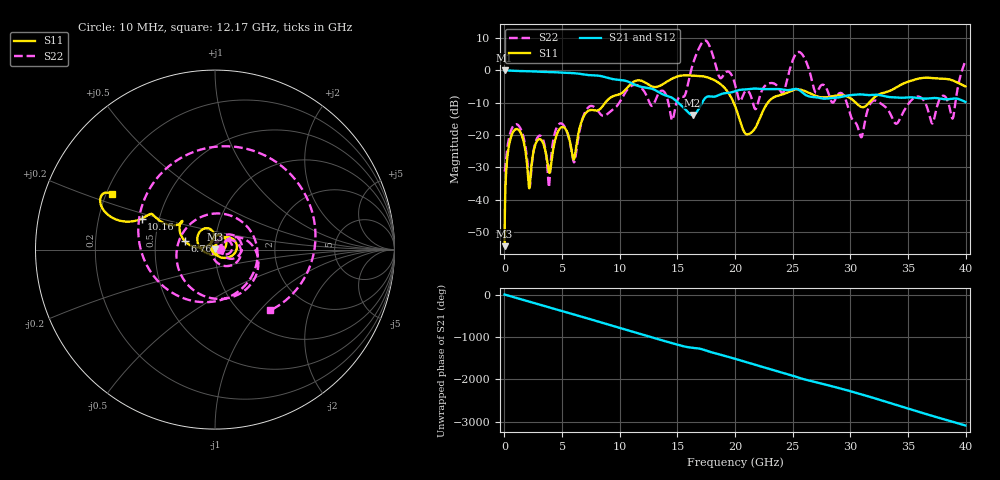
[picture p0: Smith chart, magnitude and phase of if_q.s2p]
!Keysight Technologies,N5245B,MY57181346,A.12.70.07
!Automatic Fixture Removal (AFR)
!Date: Wednesday, November 07, 2018 11:45:13 AM
!S2P File: Measurements: S11,S21,S12,S22:
# MHz S  RI  R 50
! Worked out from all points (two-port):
!   3999 points, 10 MHz to 39.99 GHz, reference 50 ohm
!   highest |S21| = 0.00 dB at 10 MHz (marker M1); lowest = -13.8 dB at 16.32 GHz (marker M2)
!   |S21| within 3 dB of the highest: start of sweep to 10.16 GHz
!   lowest |S11| = -54.4 dB at 10 MHz (marker M3), VSWR 1.00, Z = 50 + j0.189 ohm
!   |S11| at or under -10 dB: start of sweep to 8.746 GHz; 19.88 GHz to 22.85 GHz (2.965 GHz wide, 13.9 % of centre); 30.48 GHz to 31.64 GHz (1.16 GHz wide, 3.74 % of centre)
!   |S22| runs from -36.2 to 9.3 dB; largest |S21 - S12| = 1.4e-15
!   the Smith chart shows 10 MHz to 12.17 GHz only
!   S11 on the Smith chart (normalised r, x): 10 MHz: 1.00, +0.00; 6.76 GHz: 0.71, +0.07; 10.16 GHz: 0.40, +0.17; 12.17 GHz: 0.22, +0.24
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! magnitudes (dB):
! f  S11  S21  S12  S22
! 10 MHz  -54.4  0.0  0.0  -31.4
! 300 MHz  -25.3  0.0  0.0  -22.8
! 840 MHz  -18.6  -0.2  -0.2  -16.9
! 2.19 GHz  -35.8  -0.3  -0.3  -36.1
! 2.94 GHz  -21.4  -0.4  -0.4  -20.4
! 3.85 GHz  -31.4  -0.5  -0.5  -36.2
! 4.63 GHz  -19.1  -0.6  -0.6  -17.0
! 6.03 GHz  -27.5  -0.9  -0.9  -28.5
! 6.68 GHz  -15.9  -1.1  -1.1  -16.2
! 6.76 GHz  -15.1  -1.2  -1.2  -15.1
! 10.16 GHz  -7.1  -3.0  -3.0  -8.8
! 12.17 GHz  -3.7  -5.3  -5.3  -6.8
! 13.34 GHz  -5.0  -6.7  -6.7  -7.3
! 14.59 GHz  -2.5  -8.6  -8.6  -15.3
! 16.32 GHz  -1.6  -13.8  -13.8  1.7
! 17.47 GHz  -2.0  -8.4  -8.4  9.2
! 20 GHz  -11.0  -6.5  -6.5  -4.3
! 26.67 GHz  -7.4  -8.2  -8.2  -3.1
! 30.92 GHz  -11.3  -7.4  -7.4  -20.6
! 33.33 GHz  -6.5  -8.2  -8.2  -12.5
! 38.87 GHz  -3.1  -8.7  -8.7  -14.9
! 39.99 GHz  -5.0  -9.8  -9.8  3.0
